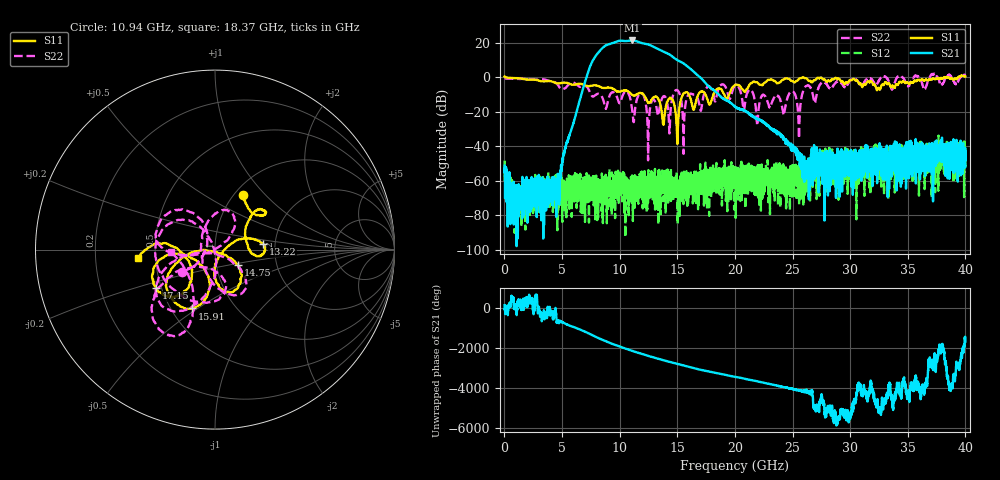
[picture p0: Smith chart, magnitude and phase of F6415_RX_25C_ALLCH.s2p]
!Keysight Technologies,N5245B,MY52451815,A.15.70.20
!Date: Wednesday, April 17, 2024 14:33:29
!Correction: S33(C  2-Port  )
!S43(C  2-Port  )
!S34(C  2-Port  )
!S44(C  2-Port  )
!S2P File: Measurements: S33, S43, S34, S44:
# Hz S  RI  R 50
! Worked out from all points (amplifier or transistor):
!   4000 points, 10 MHz to 40 GHz, reference 50 ohm
!   highest |S21| = 21.4 dB at 11.08 GHz (marker M1)
!   |S21| within 3 dB of that: 8.756 GHz to 12.73 GHz (3.97 GHz wide, 37 % of centre)
!   unconditionally stable (mu >= 1): 139.6 MHz to 25.88 GHz; 25.98 GHz to 32.69 GHz; 34.55 GHz to 35.51 GHz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
!   at 6.67 GHz: K = 1771.48, MAG = -6.1 dB, |S12| = -68.7 dB
!   at 20.01 GHz: K = 2380.76, MAG = -13.4 dB, |S12| = -63.8 dB
!   at 40 GHz: K = 472.70, MSG = 1.3 dB, |S12| = -46.0 dB
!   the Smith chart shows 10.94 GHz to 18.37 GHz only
!   S11 on the Smith chart (normalised r, x): 10.94 GHz: 1.10, +0.75; 13.22 GHz: 1.73, +0.12; 14.75 GHz: 1.27, -0.22; 15.91 GHz: 0.63, -0.47; 17.15 GHz: 0.47, -0.24; 18.37 GHz: 0.40, -0.05
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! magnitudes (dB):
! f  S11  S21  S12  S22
! 10 MHz  0.4  -51.3  -48.4  -0.7
! 930 MHz  -0.5  -63.8  -66.6  -0.8
! 4.58 GHz  -3.6  -60.0  -64.7  -3.9
! 6.68 GHz  -3.9  -9.7  -68.1  -5.4
! 8.32 GHz  -5.6  15.8  -59.8  -10.0
! 10.94 GHz  -9.4  21.4  -70.9  -13.0
! 11.08 GHz  -10.2  21.4  -57.0  -18.9
! 11.85 GHz  -9.2  20.0  -55.5  -9.3
! 12.45 GHz  -14.6  19.2  -65.2  -39.5
! 13.22 GHz  -11.4  16.8  -62.5  -18.4
! 13.34 GHz  -12.6  16.4  -54.3  -22.2
! 14.75 GHz  -16.3  11.1  -63.8  -8.3
! 15.03 GHz  -31.4  9.9  -85.2  -7.6
! 15.54 GHz  -9.3  8.1  -60.3  -44.4
! 15.91 GHz  -9.1  6.3  -64.3  -10.7
! 17.15 GHz  -8.1  -1.1  -54.3  -15.3
! 18.37 GHz  -7.3  -8.6  -59.7  -12.2
! 20.01 GHz  -4.4  -17.0  -63.8  -4.9
! 21.94 GHz  -2.9  -23.9  -61.8  -27.9
! 26.67 GHz  -2.9  -41.1  -48.8  -7.7
! 33.34 GHz  -3.6  -46.6  -45.3  -2.1
! 40 GHz  0.4  -43.4  -46.0  1.2
